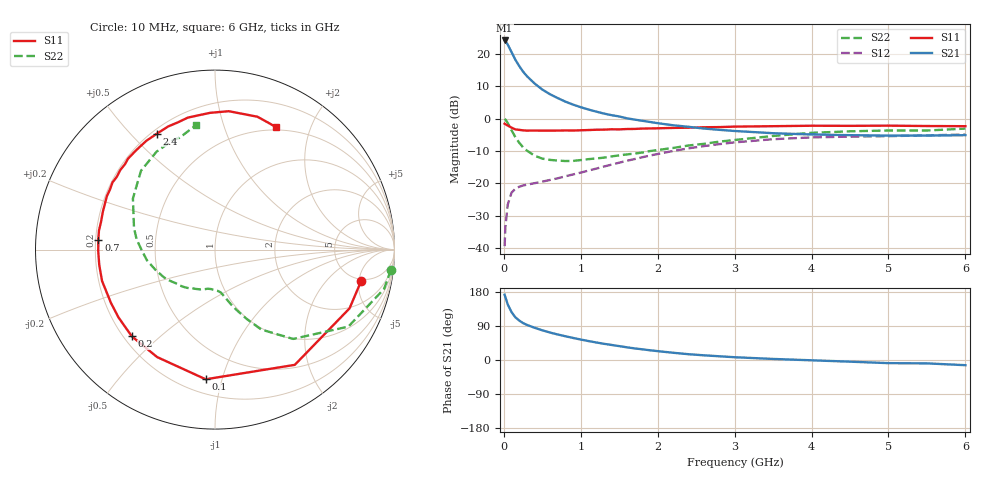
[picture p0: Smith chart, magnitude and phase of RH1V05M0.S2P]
! SIEMENS Small Signal Semiconductors
! BFR106
! Si NPN RF Bipolar Junction Transistor in SOT23
! VCE = 1 V  IC = 5 mA
! Common Emitter S-Parameters:  August  1996
# GHz  S  MA  R  50
!  f  S11  S21  S12  S22
! GHz  MAG  ANG  MAG  ANG  MAG  ANG  MAG  ANG
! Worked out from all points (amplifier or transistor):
!   36 points, 10 MHz to 6 GHz, reference 50 ohm
!   highest |S21| = 24.1 dB at 10 MHz (marker M1)
!   |S21| within 3 dB of that: start of sweep to 87.14 MHz
!   unconditionally stable (mu >= 1): 590.6 MHz to 2.984 GHz; 3.048 GHz to end of sweep
!   at 250 MHz: K = 0.52, MSG = 17.6 dB, |S12| = -20.7 dB
!   at 1.4 GHz: K = 1.18, MAG = 5.1 dB, |S12| = -14.2 dB
!   at 6 GHz: K = 1.03, MAG = -1.1 dB, |S12| = -4.9 dB
!   S11 on the Smith chart (normalised r, x): 10 MHz: 4.76, -5.40; 100 MHz: 0.29, -0.89; 200 MHz: 0.23, -0.41; 700 MHz: 0.21, +0.04; 2.4 GHz: 0.22, +0.60; 6 GHz: 0.47, +1.51
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0.01  0.8333 -12.0  16.07 172.3  0.0107 85.1  0.9867 -6.5
0.02  0.818 -23.6  15.81 166.0  0.0211 77.9  0.9671 -13.1
0.05  0.781 -55.3  13.92 147.0  0.0466 62.3  0.858 -30.0
0.1  0.7244 -94.1  10.61 126.4  0.0719 46.6  0.6614 -48.8
0.15  0.6801 -118.3  8.083 112.6  0.0824 37.7  0.515 -59.9
0.2  0.6695 -133.8  6.474 104.1  0.0885 34.2  0.4239 -65.5
0.25  0.6572 -144.9  5.31 97.4  0.0927 32.4  0.3587 -70.2
0.3  0.6513 -152.9  4.515 92.7  0.0953 32.4  0.3201 -73.5
0.4  0.6531 -164.5  3.476 85.0  0.1005 33.5  0.267 -78.7
0.5  0.6506 -172.5  2.806 78.4  0.1062 35.2  0.2406 -82.4
0.6  0.6507 -179.3  2.376 72.5  0.1127 37.8  0.2299 -86.6
0.7  0.6523 175.1  2.072 67.3  0.1195 40.6  0.2247 -91.5
0.9  0.6535 166.3  1.641 58.2  0.1371 45.3  0.2217 -100.5
1.1  0.6648 157.2  1.379 50.0  0.1573 48.4  0.2362 -110.0
1.3  0.6741 150.2  1.195 42.8  0.1815 50.4  0.2492 -119.7
1.6  0.6893 139.9  1.009 33.5  0.223 51.3  0.2796 -134.2
2.2  0.7168 122.3  0.788 19.1  0.3159 46.4  0.3517 -161.7
2.4  0.7226 116.5  0.746 15.3  0.3468 43.6  0.3836 -171.0
3.5  0.7624 92.1  0.594 2.8  0.48 24.2  0.5387 148.1
4.5  0.7719 77.7  0.554 -4.4  0.526 7.7  0.6356 120.8
5.5  0.7669 67.3  0.546 -8.9  0.5505 -2.0  0.6535 107.6
6  0.7622 63.5  0.554 -13.7  0.5665 -8.7  0.7001 98.9
